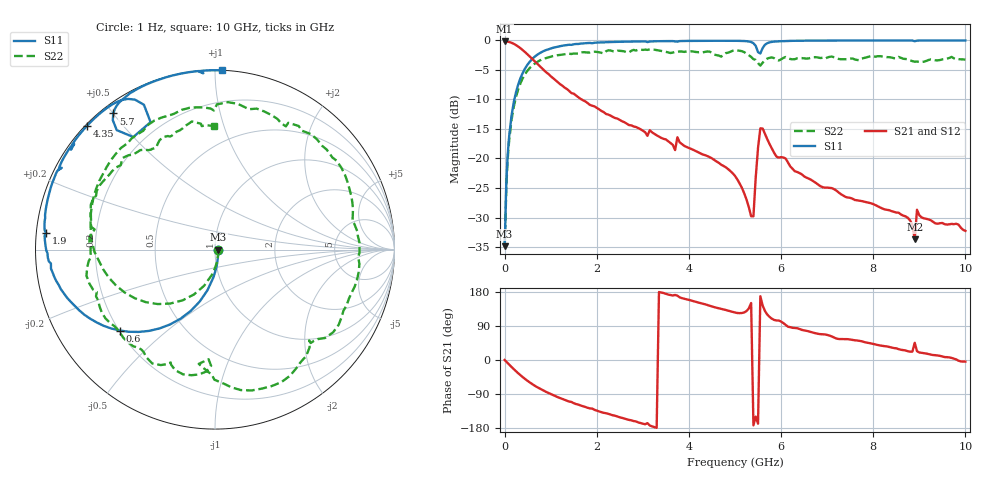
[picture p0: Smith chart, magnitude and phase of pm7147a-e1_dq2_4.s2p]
# GHz S DB R 50
! S-Parameters data
! Freq  dbS11  angS11  dbS21  angS21  dbS12  angS12  dbS22  angS22
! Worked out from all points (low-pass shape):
!   279 points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, 1 Hz to 10 GHz, reference 50 ohm
!   highest |S21| = -0.16 dB at 251.2 Hz (marker M1); lowest = -33.7 dB at 8.9 GHz (marker M2)
!   |S21| within 3 dB of the highest: start of sweep to 603.4 MHz
!   lowest |S11| = -34.9 dB at 251.2 Hz (marker M3), VSWR 1.04, Z = 51.8 - j3.42e-05 ohm
!   |S11| at or under -10 dB: start of sweep to 212.4 MHz
!   |S22| runs from -34.9 to -1.5 dB; largest |S21 - S12| = 0
!   S11 on the Smith chart (normalised r, x): 1 Hz: 1.04, -0.00; 600 MHz: 0.20, -0.35; 1.9 GHz: 0.03, +0.05; 4.35 GHz: 0.00, +0.41; 5.7 GHz: 0.03, +0.50; 10 GHz: 0.00, +1.04
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1e-09  -34.86 -0.0  -0.16 -0.0  -0.16 -0.0  -34.86 -0.0
2.512e-07  -34.86 -0.0  -0.16 -0.0  -0.16 -0.0  -34.86 -0.0
0.05011872  -21.88 -81.9  -0.19 -6.2  -0.19 -6.2  -22.57 -83.1
0.15  -12.75 -100.5  -0.40 -18.4  -0.40 -18.4  -13.49 -106.9
0.35  -6.27 -120.9  -1.36 -40.8  -1.36 -40.8  -7.14 -136.3
0.6  -3.14 -139.7  -3.13 -63.7  -3.13 -63.7  -4.27 -165.2
1.05  -1.25 -161.8  -6.38 -92.7  -6.38 -92.7  -2.65 156.6
1.7  -0.50 178.9  -10.14 -121.8  -10.14 -121.8  -2.00 115.0
1.9  -0.48 174.3  -11.07 -128.2  -11.07 -128.2  -1.94 103.4
2.75  -0.19 158.6  -14.39 -159.2  -14.39 -159.2  -1.77 60.0
3.35  -0.13 149.5  -16.30 179.4  -16.30 179.4  -1.72 23.9
4.35  -0.07 135.9  -19.43 147.0  -19.43 147.0  -1.95 -28.0
5.05  -0.07 126.4  -23.55 124.1  -23.55 124.1  -1.69 -67.6
5.4  -0.47 118.1  -29.79 -172.3  -29.79 -172.3  -3.17 -91.6
5.55  -2.22 126.0  -14.89 168.2  -14.89 168.2  -4.27 -93.3
5.7  -0.47 126.8  -16.73 120.0  -16.73 120.0  -3.08 -97.2
6.7  -0.03 113.0  -23.86 72.0  -23.86 72.0  -2.85 -147.9
8.35  -0.01 98.9  -28.78 34.3  -28.78 34.3  -2.84 142.7
8.75  -0.01 95.9  -30.05 23.2  -30.05 23.2  -3.19 126.9
8.9  -0.13 93.8  -33.72 45.5  -33.72 45.5  -3.60 122.5
8.95  -0.04 95.2  -28.69 23.2  -28.69 23.2  -3.58 122.2
10  -0.01 87.8  -32.26 -4.3  -32.26 -4.3  -3.26 90.4
